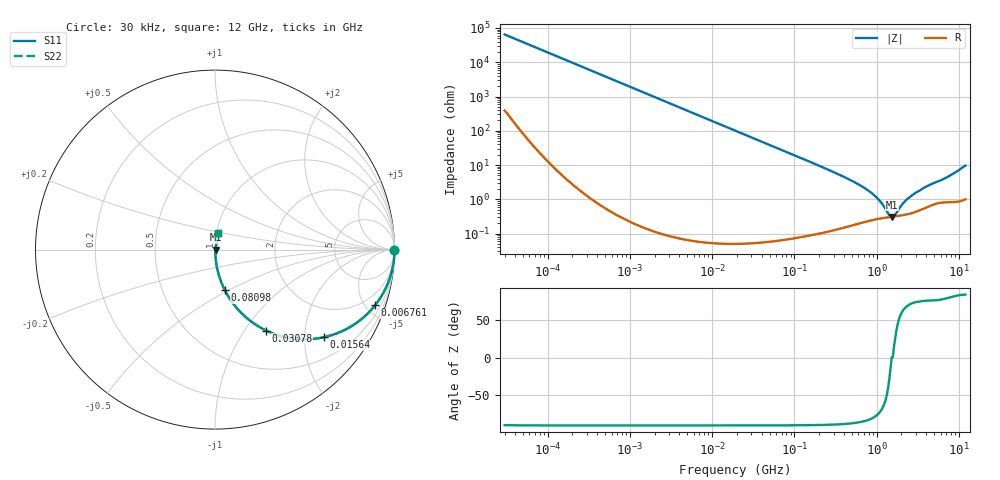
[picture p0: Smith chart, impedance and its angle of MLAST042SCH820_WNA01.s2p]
! MLAST042SCH820_WNA01  S-PARAMETER MODEL  ( General Type )
! Model Generated by TAIYO YUDEN Corporation (http://www.ty-top.com)
! Version 1.0
! TAIYO YUDEN Control No. 150820
! Copyright(c) 2015 TAIYO YUDEN CO.,LTD. All Rights Reserved.
! Product Description (link to TY-COMPAS)
! https://ds.yuden.co.jp/TYCOMPAS/or/detail?pn=MLAST042SCH820JWNA01&u=M
! Products Name : Multilayer Ceramic Capacitors
! Characteristics :
!  Capacitance : 82 pF , Rated Voltage : 25V , TCC : CH / C0H
!  Case Size : 0.4 x 0.2 / 0.016 x 0.008 [mm/inch] , Thickness : 0.2 / 0.008 [mm/inch]
!  (Conditions: Temperature = 25 degC , DC Bias Current/Voltage = 0A / 0V)
! External Node Assignments :
!  1  o---| |---o  2
! GND o---------o GND
! Frequency Range : 0.03MHz  -  12000MHz  [ 401 STEP ]
# MHz S RI R 50
! Freq[MHz].  S11 Real  S11 Imag  S21 Real  S21 Imag  S12 Real  S12 Imag  S22 Real  S22 Imag
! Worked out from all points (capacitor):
!   401 points, 30 kHz to 12 GHz, reference 50 ohm
!   read as one part in series: C = 82 pF near 32 kHz
!   lowest |Z| = 306 mohm at 1.524 GHz (marker M1)
!   series resonance near 1.523 GHz, so ESL is about 130 pH
!   S11 on the Smith chart (normalised r, x): 30 kHz: open; 6.761 MHz: 1.00, -5.74; 15.64 MHz: 1.00, -2.48; 30.78 MHz: 1.00, -1.26; 80.98 MHz: 1.00, -0.48; 12 GHz: 1.02, +0.19
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0.03  1 -0.00155  1.16e-05 0.00155  1.16e-05 0.00155  1 -0.00155
0.260295  0.9998 -0.0134  0.000183 0.0134  0.000183 0.0134  0.9998 -0.0134
2.258455  0.9866 -0.1148  0.0134 0.1148  0.0134 0.1148  0.9866 -0.1148
6.760619  0.8917 -0.3106  0.1083 0.3106  0.1083 0.3106  0.8917 -0.3106
10.28143  0.7808 -0.4136  0.2192 0.4136  0.2192 0.4136  0.7808 -0.4136
15.63581  0.6063 -0.4884  0.3937 0.4884  0.3937 0.4884  0.6063 -0.4884
18.97367  0.5113 -0.4996  0.4887 0.4996  0.4887 0.4996  0.5113 -0.4996
30.77716  0.2845 -0.4508  0.7155 0.4508  0.7155 0.4508  0.2845 -0.4508
48.33933  0.1389 -0.3452  0.8611 0.3452  0.8611 0.3452  0.1389 -0.3452
80.98098  0.0546 -0.2258  0.9454 0.2258  0.9454 0.2258  0.0546 -0.2258
164.6252  0.0143 -0.1148  0.9857 0.1148  0.9857 0.1148  0.0143 -0.1148
433.1624  0.00324 -0.041  0.9968 0.041  0.9968 0.041  0.00324 -0.041
749.4426  0.00261 -0.0195  0.9974 0.0195  0.9974 0.0195  0.00261 -0.0195
1068.55  0.00279 -0.00914  0.9972 0.00914  0.9972 0.00914  0.00279 -0.00914
1428.372  0.00299 -0.00159  0.997 0.00159  0.997 0.00159  0.00299 -0.00159
1523.532  0.00305 1.09e-05  0.997 -1.09e-05  0.997 -1.09e-05  0.00305 1.09e-05
1678.29  0.00316 0.0015  0.9968 -0.0015  0.9968 -0.0015  0.00316 0.0015
2172.242  0.00354 0.00749  0.9965 -0.00749  0.9965 -0.00749  0.00354 0.00749
2811.574  0.00425 0.0134  0.9958 -0.0134  0.9958 -0.0134  0.00425 0.0134
4008.724  0.00622 0.0225  0.9938 -0.0225  0.9938 -0.0225  0.00622 0.0225
7163.064  0.00996 0.0424  0.99 -0.0424  0.99 -0.0424  0.00996 0.0424
12000  0.0187 0.093  0.9813 -0.093  0.9813 -0.093  0.0187 0.093
